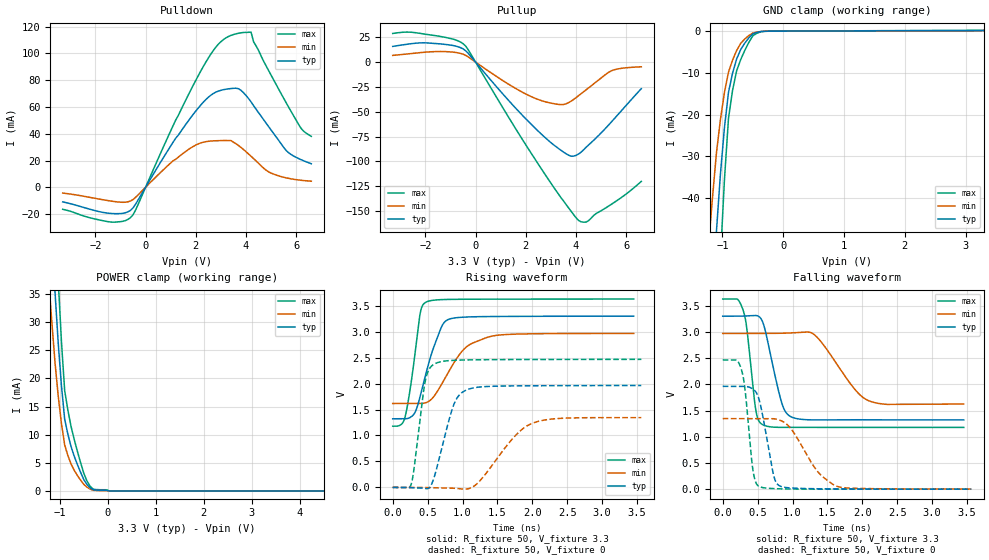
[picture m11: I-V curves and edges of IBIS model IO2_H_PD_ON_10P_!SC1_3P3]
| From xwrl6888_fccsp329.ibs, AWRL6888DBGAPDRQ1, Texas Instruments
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|   Model Cell IO2_H_PD_ON_10P_!SC1_3P3
|IO2_H_PD_ON_10P_!SC1_3P3
[Model]   IO2_H_PD_ON_10P_!SC1_3P3
Model_type   I/O
Polarity   Non-Inverting
Enable   Active-Low
Vinl =  0.8V
Vinh =  2V
Cref =  15pF
Rref =  100.0000M
Vref =  0V
Vmeas =  1.65
|   typ   min   max
C_comp   2.157014p   1.997104p   2.250886p
[Model Spec]
Vinl   0.8V   0.8V   0.8V
Vinh   2V   2V   2V
[Temperature Range]   25   125   -40
[Voltage Range]   3.3   2.97   3.63
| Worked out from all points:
|   slope of the pulldown table from 0 to 0.495 V, typ, clamps not added: 31.8 ohm
|   slope of the pullup table from 0 to 0.495 V, typ, clamps not added: 33.3 ohm
|   GND clamp passes 1 mA (typ) near -0.52 V on its own axis
|   POWER clamp passes 1 mA (typ) near -0.42 V on its own axis
|   rising waveform, R_fixture 50, V_fixture 3.3: 20-80 % time 258ps typ, 391ps min, 146ps max; typ from 1.32 V to 3.3 V
|   rising waveform, R_fixture 50, V_fixture 0: 20-80 % time 233ps typ, 479ps min, 138ps max; typ from 0 V to 1.96 V
|   falling waveform, R_fixture 50, V_fixture 3.3: 20-80 % time 199ps typ, 427ps min, 119ps max; typ from 3.3 V to 1.32 V
|   falling waveform, R_fixture 50, V_fixture 0: 20-80 % time 162ps typ, 386ps min, 107ps max; typ from 1.96 V to 0 V
| Where Nom  PVT is Nominal Process, 3.3V, 25C
|   Fast PVT is Strong Process,  3.63V, -40C
|   Slow PVT is Weak Process,   2.97V, 125C
[POWER_clamp]
|   voltage   I(typ)   I(min)   I(max)
-3.3V     446.9mA    419.5mA    603.9mA
-1.233V   56.59mA    37.53mA    80.37mA
-1.167V   45.68mA    29.91mA    65.17mA
-1.1V     35.14mA    22.67mA    50.36mA
-1.033V   26.13mA    16.78mA    37.31mA
-966.7mV  18.67mA    11.95mA    26.46mA
-900mV    12.76mA    8.172mA    17.82mA
-833.3mV  10.07mA    6.29mA     14.35mA
-566.7mV  3.276mA    1.904mA    4.983mA
-366.7mV  519.9uA    307.2uA    792.3uA
33.33mV   0A         0A         0A
6.6V      0A         0A         0A
[Pulldown]
|   voltage   I(typ)   I(min)   I(max)
-3.3V     -10.92mA   -4.307mA   -16.45mA
-1.4V     -19.52mA   -10.22mA   -25.94mA
-600mV    -17.22mA   -10.25mA   -22.66mA
1.1V      33.8mA     19.88mA    46.22mA
2.1V      59.3mA     32.44mA    83.48mA
2.9V      71.86mA    34.84mA    107mA
3.5V      73.95mA    33.66mA    114.2mA
4.2V      63.8mA     23.19mA    116mA
4.9V      45.33mA    11.53mA    87.2mA
5.6V      27.47mA    7.046mA    63.1mA
6.2V      20.56mA    5.221mA    43.87mA
6.6V      17.6mA     4.555mA    38.05mA
[Pullup]
|   voltage   I(typ)   I(min)   I(max)
-3.3V     15.77mA    6.741mA    28.8mA
-1.9V     19.23mA    10.15mA    27.67mA
-900mV    16.69mA    10.02mA    23.17mA
-400mV    11.53mA    6.853mA    16.25mA
1.3V      -38.16mA   -22.04mA   -54.89mA
2.3V      -64.7mA    -35.66mA   -95.04mA
3.4V      -88.76mA   -42.82mA   -136.4mA
3.8V      -94.64mA   -39.36mA   -150mA
4.1V      -92.53mA   -33.79mA   -159.3mA
4.4V      -85.77mA   -27.94mA   -161mA
5.4V      -60.46mA   -8.849mA   -143.2mA
6.6V      -26.71mA   -4.741mA   -120mA
[GND_clamp]
|   voltage   I(typ)   I(min)   I(max)
-3.3V     -787.2mA   -607.8mA   -1.235A
-1.233V   -85.66mA   -52.14mA   -138.8mA
-1.167V   -66.47mA   -40.37mA   -107.7mA
-1.1V     -48.25mA   -29.37mA   -77.99mA
-1.033V   -34.28mA   -21.19mA   -54.56mA
-966.7mV  -23.07mA   -14.67mA   -35.51mA
-900mV    -14.62mA   -9.792mA   -20.84mA
-833.3mV  -10.07mA   -6.938mA   -14.17mA
-700mV    -4.435mA   -2.939mA   -6.836mA
-500mV    -641.2uA   -454.5uA   -1.12mA
-300mV    -31.62uA   -32.73uA   -44.27uA
3.3V      108.6uA    159.4uA    198.5uA
[Ramp]
| variable   typ   min   max
dV/dt_f  1.1954816/0.20074978n 0.83576296/0.44363752n  1.4751037/0.11965581n
dV/dt_r  1.1916349/0.23568191n 0.82814892/0.49061137n  1.4892937/0.13872759n
R_load = 50
[Rising Waveform]
R_fixture = 50
V_fixture = 3.3
V_fixture_min = 2.97
V_fixture_max = 3.63
|   time   V(typ)   V(min)   V(max)
0s        1.321V     1.616V     1.179V
177.6ps   1.321V     1.616V     1.358V
303.9ps   1.411V     1.616V     2.409V
389.3ps   1.733V     1.616V     3.322V
475.1ps   2.187V     1.631V     3.566V
695.1ps   3.08V      1.973V     3.616V
824.7ps   3.247V     2.281V     3.621V
1.069ns   3.282V     2.719V     3.624V
1.434ns   3.291V     2.916V     3.625V
3.453ns   3.297V     2.965V     3.627V
[Rising Waveform]
R_fixture = 50
V_fixture = 0
V_fixture_min = 0
V_fixture_max = 0
|   time   V(typ)   V(min)   V(max)
0s        0V         0V         0V
263ps     -5.429mV   0V         55.93mV
302.5ps   -7.292mV   0V         330.3mV
465.3ps   -20.65mV   -2.403mV   2.039V
538ps     15.37mV    -3.759mV   2.309V
607.8ps   257.9mV    -5.571mV   2.384V
871.4ps   1.58V      -15.22mV   2.447V
1.058ns   1.877V     -31.71mV   2.455V
2.001ns   1.957V     1.234V     2.463V
3.562ns   1.962V     1.344V     2.465V
[Falling Waveform]
R_fixture = 50
V_fixture = 3.3
V_fixture_min = 2.97
V_fixture_max = 3.63
|   time   V(typ)   V(min)   V(max)
0s        3.299V     2.97V      3.626V
296.4ps   3.299V     2.97V      3.397V
344.8ps   3.305V     2.97V      3.071V
476.3ps   3.312V     2.97V      1.493V
574.8ps   3.182V     2.97V      1.228V
840.1ps   1.67V      2.974V     1.179V
984ps     1.377V     2.98V      1.179V
1.328ns   1.32V      2.929V     1.179V
2.096ns   1.323V     1.684V     1.178V
3.453ns   1.321V     1.624V     1.178V
[Falling Waveform]
R_fixture = 50
V_fixture = 0
V_fixture_min = 0
V_fixture_max = 0
|   time   V(typ)   V(min)   V(max)
0s        1.961V     1.346V     2.465V
269.2ps   1.961V     1.346V     2.276V
320ps     1.96V      1.346V     1.899V
432.6ps   1.911V     1.346V     366.2mV
521.1ps   1.709V     1.346V     52.16mV
729.8ps   262.9mV    1.343V     10.73mV
824.7ps   56.8mV     1.312V     6.105mV
1.374ns   6.947mV    314mV      0V
1.63ns    4.837mV    58.06mV    0V
3.562ns   0V         2.766mV    0V
